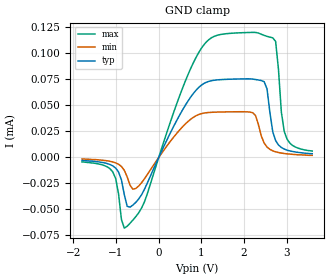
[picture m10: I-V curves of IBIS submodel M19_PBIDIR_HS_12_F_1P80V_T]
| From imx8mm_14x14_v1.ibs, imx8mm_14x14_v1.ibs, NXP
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| Submodel
[Submodel]  M19_PBIDIR_HS_12_F_1P80V_T
Submodel_type Dynamic_clamp
[GND Clamp]
| Voltage   I(typ)   I(min)   I(max)
-1.8V     -2.889uA   -1.55uA    -4.319uA
-1.076V   -8.106uA   -4.321uA   -14.01uA
-874.1mV  -21.63uA   -8.65uA    -59.68uA
-739.7mV  -46.95uA   -18.71uA   -66.13uA
-470.7mV  -39.96uA   -27.48uA   -53.23uA
931mV     67.05uA    41.19uA    100.4uA
1.867V    75.45uA    43.96uA    119.8uA
2.271V    74.93uA    40.29uA    120.2uA
2.472V    72.83uA    13.85uA    117.4uA
2.741V    16.22uA    5.424uA    111.6uA
2.943V    8.076uA    3.815uA    25.08uA
3.6V      3.604uA    2.027uA    6.162uA
